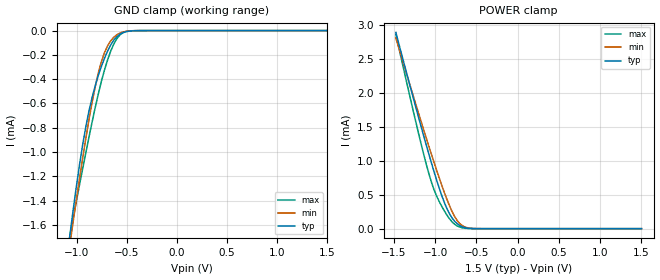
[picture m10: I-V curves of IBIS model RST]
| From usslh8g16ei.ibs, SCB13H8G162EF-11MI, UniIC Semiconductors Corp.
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|   Model RST
[Model] RST
Model_type Input
Polarity   Non-Inverting
Enable   Active-High
Vinl =  0.300V
Vinh =  1.200V
C_comp   0.101pF   76.222fF   0.113pF
C_comp_power_clamp   39.982fF   33.446fF   48.055fF
C_comp_gnd_clamp   64.979fF   36.239fF   67.109fF
[Model Spec]
Vinh   1.200V   1.026V   1.260V
Vinl   0.300V   0.257V   0.315V
[Temperature Range]   45.000   95.000   -40.000
[Voltage Range]   1.500V   1.283V   1.575V
[C Comp Corner]
C_comp_power_clamp   33.446fF   39.982fF   48.055fF
C_comp_gnd_clamp   67.109fF   36.239fF   64.979fF
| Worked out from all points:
|   GND clamp passes 1 mA (typ) near -0.95 V on its own axis
|   POWER clamp passes 1 mA (typ) near -1.05 V on its own axis
[GND_clamp]
|Voltage   I(typ)   I(min)   I(max)
-1.5V     -4.711mA   -4.355mA   -5.13mA
-1.066V   -1.656mA   -1.736mA   -1.672mA
-1.035V   -1.461mA   -1.559mA   -1.532mA
-942mV    -937.4uA   -1.048mA   -1.135mA
-849mV    -553.6uA   -594.1uA   -756.1uA
-787mV    -372.4uA   -351.5uA   -524.2uA
-725mV    -228.7uA   -182.7uA   -326uA
-663mV    -119.4uA   -85.26uA   -170.5uA
-601mV    -49.81uA   -34.44uA   -66.38uA
-539mV    -16.69uA   -11.31uA   -17.39uA
-446mV    -2.392uA   -1.689uA   -1.296uA
1.5V      0A         0A         0A
[POWER_clamp]
|Voltage   I(typ)   I(min)   I(max)
-1.476V   2.894mA    2.812mA    2.865mA
-1.197V   1.625mA    1.687mA    1.386mA
-1.104V   1.219mA    1.323mA    935.8uA
-1.042V   957.4uA    1.086mA    675.5uA
-980mV    709.1uA    854.8uA    475.2uA
-887mV    381.5uA    528.9uA    259.3uA
-825mV    216.9uA    335.6uA    144.5uA
-763mV    108.7uA    177.7uA    64.17uA
-732mV    72.5uA     118.4uA    39.23uA
-670mV    26.52uA    43.96uA    12.12uA
-546mV    1.464uA    3.136uA    422.4nA
1.5V      0A         0A         0A
